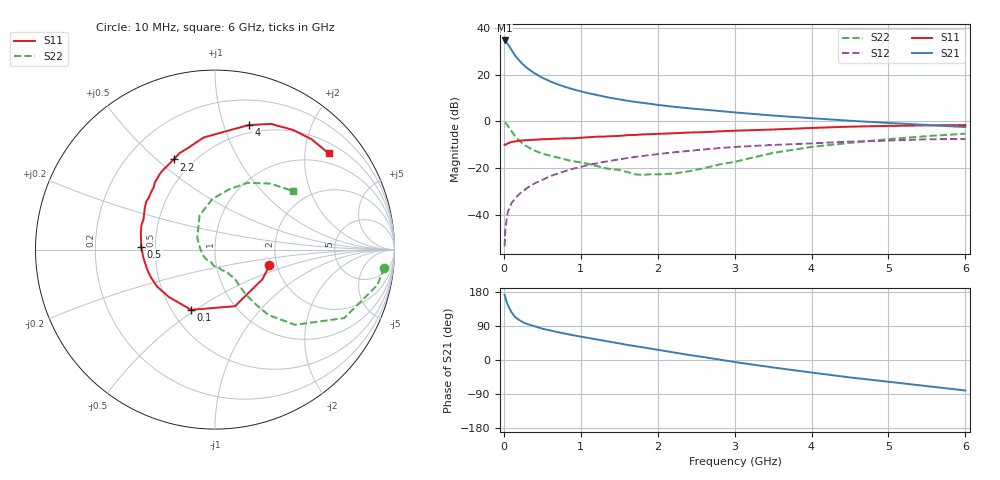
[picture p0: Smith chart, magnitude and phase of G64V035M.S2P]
! SIEMENS Small Signal Semiconductors
! BFG193
! Si NPN RF Bipolar Junction Transistor in SOT223
! VCE = 4 V  IC = 35 mA
! Common Emitter S-Parameters:  August  1996
# GHz  S  MA  R  50
!  f  S11  S21  S12  S22
! GHz  MAG  ANG  MAG  ANG  MAG  ANG  MAG  ANG
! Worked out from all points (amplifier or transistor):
!   36 points, 10 MHz to 6 GHz, reference 50 ohm
!   highest |S21| = 34.7 dB at 10 MHz (marker M1)
!   |S21| within 3 dB of that: start of sweep to 79.22 MHz
!   unconditionally stable (mu >= 1): 503.4 MHz to 2.45 GHz
!   at 250 MHz: K = 0.86, MSG = 27.1 dB, |S12| = -29.9 dB
!   at 1.4 GHz: K = 1.04, MAG = 12.2 dB, |S12| = -16.9 dB
!   at 6 GHz: K = 0.89, MSG = 2.6 dB, |S12| = -7.6 dB
!   S11 on the Smith chart (normalised r, x): 10 MHz: 1.83, -0.36; 100 MHz: 0.62, -0.48; 500 MHz: 0.42, +0.02; 2.2 GHz: 0.39, +0.57; 4 GHz: 0.42, +1.22; 6 GHz: 0.74, +2.54
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0.01  0.3158 -16.2  54.08 171.9  0.0021 88.9  0.9491 -6.1
0.02  0.3118 -31.9  52.69 165.0  0.0049 79.8  0.9253 -12.4
0.05  0.3346 -70.6  45.68 145.4  0.0111 72.0  0.8151 -27.9
0.1  0.361 -111.7  33.77 125.7  0.0177 65.2  0.612 -43.2
0.15  0.3687 -134.5  25.22 112.8  0.0225 63.6  0.4716 -50.7
0.2  0.3829 -147.6  20.09 105.5  0.0275 64.9  0.3877 -53.1
0.25  0.3889 -156.4  16.46 99.6  0.032 65.3  0.3251 -54.8
0.3  0.394 -163.4  13.95 95.3  0.0368 66.1  0.2882 -55.7
0.4  0.4021 -174.0  10.67 88.9  0.0466 66.9  0.2344 -55.9
0.5  0.4115 177.8  8.586 82.8  0.0555 66.1  0.2028 -55.9
0.6  0.4161 171.9  7.22 78.2  0.066 65.3  0.1835 -56.9
0.7  0.4244 166.8  6.218 73.6  0.0757 64.3  0.1673 -59.0
0.8  0.4313 161.7  5.437 69.4  0.0857 62.8  0.1512 -60.8
1.1  0.455 149.4  3.995 58.1  0.1153 58.1  0.1217 -71.1
1.6  0.503 131.7  2.766 40.1  0.162 47.5  0.0822 -100.4
2.2  0.5525 114.6  2.053 20.3  0.2154 34.3  0.0754 -161.9
2.8  0.6074 99.7  1.661 1.2  0.2662 20.5  0.1183 146.5
3.5  0.6665 83.7  1.326 -19.7  0.3111 3.4  0.2098 114.1
4  0.7188 74.9  1.164 -33.1  0.3354 -6.3  0.2822 93.1
4.5  0.7671 65.9  1.027 -46.0  0.3661 -16.5  0.3448 76.8
5.5  0.817 48.8  0.834 -68.9  0.4114 -39.8  0.4801 50.0
6  0.8298 40.3  0.752 -80.5  0.4174 -53.2  0.5416 37.1
